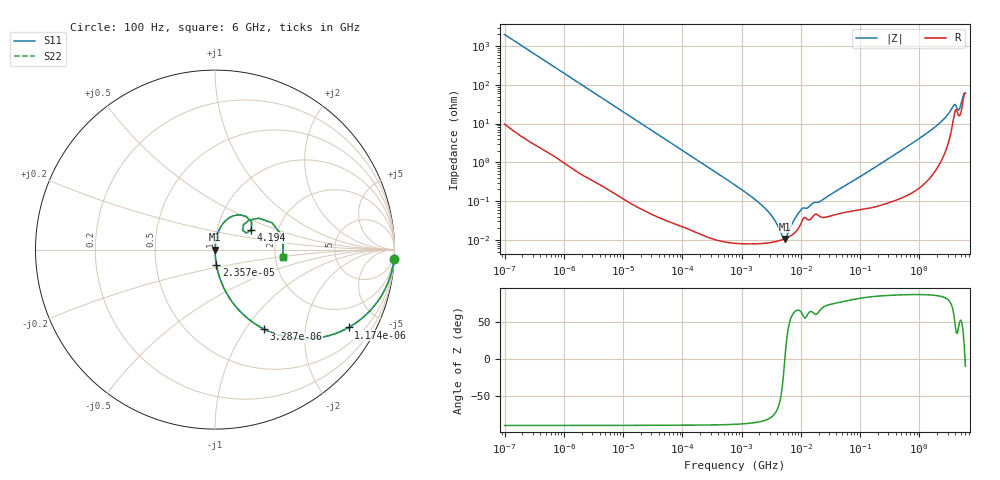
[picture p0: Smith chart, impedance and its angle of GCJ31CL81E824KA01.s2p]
!Murata Part Number: GCJ31CL81E824KA01
!These Parameters are Measured in Series Mode Connection
!Data Generated on Mar 13, 2026
!  o--ll--o
!Port1  Port2
!  o------o
!Operation Temp=25[degC], DC Bias Voltage=0[V]
!Freq. Start=100[Hz] Stop=6[GHz] 401[Steps]
# Hz S RI R 50
!Freq.(Hz) S11(Real) S11(Imag) S21(Real) S21(Imag) S12(Real) S12(Imag) S22(Real) S22(Imag)
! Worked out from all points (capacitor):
!   401 points, 100 Hz to 6 GHz, reference 50 ohm
!   read as one part in series: C = 798 nF near 109 Hz
!   lowest |Z| = 10.6 mohm at 5.312 MHz (marker M1)
!   series resonance near 5.378 MHz, so ESL is about 1.1 nH
!   S11 on the Smith chart (normalised r, x): 100 Hz: 1, -40; 1.174 kHz: 1.02, -3.42; 3.287 kHz: 1.01, -1.23; 23.57 kHz: 1.00, -0.17; 4.194 GHz: 1.46, +0.34; 6 GHz: 2.21, -0.21
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100  0.9972 -0.05  0.00275 0.05  0.00275 0.05  0.9972 -0.05
479  0.9448 -0.226  0.0552 0.226  0.0552 0.226  0.9448 -0.226
1174  0.7443 -0.4339  0.2557 0.4339  0.2557 0.4339  0.7443 -0.4339
2008  0.5005 -0.4976  0.4995 0.4976  0.4995 0.4976  0.5005 -0.4976
3287  0.2739 -0.4434  0.7261 0.4434  0.7261 0.4434  0.2739 -0.4434
7358  0.0712 -0.2544  0.9288 0.2544  0.9288 0.2544  0.0712 -0.2544
23569  0.00788 -0.0852  0.9921 0.0852  0.9921 0.0852  0.00788 -0.0852
40335  0.0029 -0.0502  0.9971 0.0502  0.9971 0.0502  0.0029 -0.0502
774597  8.82e-05 -0.0026  0.9999 0.0026  0.9999 0.0026  8.82e-05 -0.0026
2594782  8.27e-05 -0.000609  0.9999 0.000609  0.9999 0.000609  8.27e-05 -0.000609
3549919  8.85e-05 -0.000328  0.9999 0.000328  0.9999 0.000328  8.85e-05 -0.000328
5311619  0.000106 -9.5e-06  0.9999 9.5e-06  0.9999 9.5e-06  0.000106 -9.5e-06
9941735  0.000254 0.000526  0.9997 -0.000526  0.9997 -0.000526  0.000254 0.000526
1.555665e7  0.00038 0.000766  0.9996 -0.000766  0.9996 -0.000766  0.00038 0.000766
2.225763e7  0.000386 0.000951  0.9996 -0.000951  0.9996 -0.000951  0.000386 0.000951
3.124326e8  0.00108 0.0128  0.9989 -0.0128  0.9989 -0.0128  0.00108 0.0128
2.34314e9  0.0226 0.1078  0.9774 -0.1078  0.9774 -0.1078  0.0226 0.1078
3.666503e9  0.1365 0.1942  0.8635 -0.1942  0.8635 -0.1942  0.1365 0.1942
4.193612e9  0.2023 0.1094  0.7977 -0.1094  0.7977 -0.1094  0.2023 0.1094
4.796499e9  0.1584 0.1377  0.8416 -0.1377  0.8416 -0.1377  0.1584 0.1377
5.245841e9  0.2448 0.1748  0.7552 -0.1748  0.7552 -0.1748  0.2448 0.1748
6e9  0.3797 -0.0403  0.6203 0.0403  0.6203 0.0403  0.3797 -0.0403
